FUNCTION_BLOCK PS_PackML_StateMachine_Auto
VAR_INPUT
	Start				: BOOL;
	Hold				: BOOL;
	UnHold				: BOOL;
	Suspend				: BOOL;
	UnSuspend			: BOOL;
	Abort				: BOOL;
	Stop				: BOOL;
	Complete			: BOOL;
	Clear				: BOOL;
	Reset				: BOOL;
	StateComplete		: BOOL;
END_VAR
VAR_OUTPUT
	Status				: WORD;

	ST_Starting			: BOOL;
	ST_Completing		: BOOL;
	ST_Resetting		: BOOL;
	ST_Holding			: BOOL;
	ST_UnHolding		: BOOL;
	ST_Suspending		: BOOL;
	ST_UnSuspending		: BOOL;
	ST_Clearing			: BOOL;
	ST_Stopping			: BOOL;
	ST_Aborting			: BOOL;

	(* State Complete*)
	ST_Execute			: BOOL;
	ST_Complete			: BOOL;
	ST_Idle				: BOOL;
	ST_Held				: BOOL;
	ST_Suspended		: BOOL;
	ST_Stopped			: BOOL;
	ST_Aborted			: BOOL;

	(* additional *)
	Error				: BOOL;
	ErrorID				: DWORD;
	ePMLState			: E_PMLState := E_PMLState.IDLE;
END_VAR
VAR
	ePMLStatePrev		: E_PMLState;
	bStateChange		: BOOL;
	StateCompletePrev	: BOOL;
END_VAR

(* check for state change *)
IF ePMLStatePrev <> ePMLState THEN
	ePMLStatePrev 	:= ePMLState;
	bStateChange	:= TRUE;
ELSE
	bStateChange	:= FALSE;
END_IF


(* change to new state if requested *)
CASE ePMLState OF
	E_PMLState.UNDEFINED:
				(* undefined state *)
				IF bStateChange THEN
					(* transient state *)
					ST_Starting		:= FALSE;
					ST_Completing	:= FALSE;
					ST_Resetting	:= FALSE;
					ST_Holding		:= FALSE;
					ST_UnHolding	:= FALSE;
					ST_Suspending	:= FALSE;
					ST_UnSuspending	:= FALSE;
					ST_Clearing		:= FALSE;
					ST_Stopping		:= FALSE;
					ST_Aborting		:= FALSE;
		
					(* final state *)
					ST_Execute		:= FALSE;
					ST_Complete		:= FALSE;
					ST_Idle			:= FALSE;
					ST_Held			:= FALSE;
					ST_Suspended	:= FALSE;
					ST_Stopped		:= FALSE;
					ST_Aborted		:= FALSE;
				END_IF
		
				IF Abort THEN
					ePMLState 		:= E_PMLState.ABORTING;
					ST_Aborting		:= TRUE;
				ELSIF Stop THEN
					ePMLState 		:= E_PMLState.STOPPING;
					ST_Stopping		:= TRUE;
				END_IF


	E_PMLState.IDLE:
				(* final state *)
		
				IF bStateChange THEN
					(* transient state *)
					ST_Starting		:= FALSE;
					ST_Completing	:= FALSE;
					ST_Resetting	:= FALSE;
					ST_Holding		:= FALSE;
					ST_UnHolding	:= FALSE;
					ST_Suspending	:= FALSE;
					ST_UnSuspending	:= FALSE;
					ST_Clearing		:= FALSE;
					ST_Stopping		:= FALSE;
					ST_Aborting		:= FALSE;
		
					(* final state *)
					ST_Execute		:= FALSE;
					ST_Complete		:= FALSE;
					ST_Idle			:= TRUE;
					ST_Held			:= FALSE;
					ST_Suspended	:= FALSE;
					ST_Stopped		:= FALSE;
					ST_Aborted		:= FALSE;
				END_IF
		
				IF Abort THEN
					ePMLState 		:= E_PMLState.ABORTING;
					ST_Idle			:= FALSE;
					ST_Aborting		:= TRUE;
				ELSIF Stop THEN
					ePMLState 		:= E_PMLState.STOPPING;
					ST_Idle			:= FALSE;
					ST_Stopping		:= TRUE;
				ELSIF Start THEN
					ePMLState 		:= E_PMLState.STARTING;
					ST_Idle			:= FALSE;
					ST_Starting		:= TRUE;
				END_IF


	E_PMLState.STARTING:
				(* transient state *)
		
				IF bStateChange THEN
					(* transient state *)
					ST_Starting		:= TRUE;
					ST_Completing	:= FALSE;
					ST_Resetting	:= FALSE;
					ST_Holding		:= FALSE;
					ST_UnHolding	:= FALSE;
					ST_Suspending	:= FALSE;
					ST_UnSuspending	:= FALSE;
					ST_Clearing		:= FALSE;
					ST_Stopping		:= FALSE;
					ST_Aborting		:= FALSE;
		
					(* final state *)
					ST_Execute		:= FALSE;
					ST_Complete		:= FALSE;
					ST_Idle			:= FALSE;
					ST_Held			:= FALSE;
					ST_Suspended	:= FALSE;
					ST_Stopped		:= FALSE;
					ST_Aborted		:= FALSE;
				END_IF
		
				IF Abort THEN
					ePMLState 		:= E_PMLState.ABORTING;
					ST_Starting		:= FALSE;
					ST_Aborting		:= TRUE;
				ELSIF Stop THEN
					ePMLState 		:= E_PMLState.STOPPING;
					ST_Starting		:= FALSE;
					ST_Stopping		:= TRUE;
				ELSIF StateComplete AND NOT StateCompletePrev THEN
					ePMLState 		:= E_PMLState.EXECUTE;
					StateCompletePrev := StateComplete;
					ST_Starting		:= FALSE;
					ST_Execute		:= TRUE;
				END_IF


	E_PMLState.EXECUTE:
				(* final state *)
		
				IF bStateChange THEN
					(* transient state *)
					ST_Starting		:= FALSE;
					ST_Completing	:= FALSE;
					ST_Resetting	:= FALSE;
					ST_Holding		:= FALSE;
					ST_UnHolding	:= FALSE;
					ST_Suspending	:= FALSE;
					ST_UnSuspending	:= FALSE;
					ST_Clearing		:= FALSE;
					ST_Stopping		:= FALSE;
					ST_Aborting		:= FALSE;
		
					(* final state *)
					ST_Execute		:= TRUE;
					ST_Complete		:= FALSE;
					ST_Idle			:= FALSE;
					ST_Held			:= FALSE;
					ST_Suspended	:= FALSE;
					ST_Stopped		:= FALSE;
					ST_Aborted		:= FALSE;
				END_IF
		
				IF Abort THEN
					ePMLState 		:= E_PMLState.ABORTING;
					ST_Execute		:= FALSE;
					ST_Aborting		:= TRUE;
				ELSIF Stop THEN
					ePMLState 		:= E_PMLState.STOPPING;
					ST_Execute		:= FALSE;
					ST_Stopping		:= TRUE;
				ELSIF Suspend THEN
					ePMLState 		:= E_PMLState.SUSPENDING;
					ST_Execute		:= FALSE;
					ST_Suspending	:= TRUE;
				ELSIF Hold THEN
					ePMLState 		:= E_PMLState.HOLDING;
					ST_Execute		:= FALSE;
					ST_Holding		:= TRUE;
				ELSIF Complete THEN
					ePMLState 		:= E_PMLState.COMPLETING;
					ST_Execute		:= FALSE;
					ST_Completing	:= TRUE;
				END_IF


	E_PMLState.COMPLETING:
				(* transient state *)
		
				IF bStateChange THEN
					(* transient state *)
					ST_Starting		:= FALSE;
					ST_Completing	:= TRUE;
					ST_Resetting	:= FALSE;
					ST_Holding		:= FALSE;
					ST_UnHolding	:= FALSE;
					ST_Suspending	:= FALSE;
					ST_UnSuspending	:= FALSE;
					ST_Clearing		:= FALSE;
					ST_Stopping		:= FALSE;
					ST_Aborting		:= FALSE;
		
					(* final state *)
					ST_Execute		:= FALSE;
					ST_Complete		:= FALSE;
					ST_Idle			:= FALSE;
					ST_Held			:= FALSE;
					ST_Suspended	:= FALSE;
					ST_Stopped		:= FALSE;
					ST_Aborted		:= FALSE;
				END_IF
		
				IF Abort THEN
					ePMLState 		:= E_PMLState.ABORTING;
					ST_Completing	:= FALSE;
					ST_Aborting		:= TRUE;
				ELSIF Stop THEN
					ePMLState 		:= E_PMLState.STOPPING;
					ST_Completing	:= FALSE;
					ST_Stopping		:= TRUE;
				ELSIF StateComplete AND NOT StateCompletePrev THEN
					ePMLState 		:= E_PMLState.COMPLETE;
					StateCompletePrev := StateComplete;
					ST_Completing	:= FALSE;
					ST_Complete		:= TRUE;
				END_IF


	E_PMLState.COMPLETE:
				(* final state *)
		
				IF bStateChange THEN
					(* transient state *)
					ST_Starting		:= FALSE;
					ST_Completing	:= FALSE;
					ST_Resetting	:= FALSE;
					ST_Holding		:= FALSE;
					ST_UnHolding	:= FALSE;
					ST_Suspending	:= FALSE;
					ST_UnSuspending	:= FALSE;
					ST_Clearing		:= FALSE;
					ST_Stopping		:= FALSE;
					ST_Aborting		:= FALSE;
		
					(* final state *)
					ST_Execute		:= FALSE;
					ST_Complete		:= TRUE;
					ST_Idle			:= FALSE;
					ST_Held			:= FALSE;
					ST_Suspended	:= FALSE;
					ST_Stopped		:= FALSE;
					ST_Aborted		:= FALSE;
				END_IF
		
				IF Abort THEN
					ePMLState 		:= E_PMLState.ABORTING;
					ST_Complete		:= FALSE;
					ST_Aborting		:= TRUE;
				ELSIF Stop THEN
					ePMLState 		:= E_PMLState.STOPPING;
					ST_Complete		:= FALSE;
					ST_Stopping		:= TRUE;
				ELSIF Reset THEN
					ePMLState 		:= E_PMLState.RESETTING;
					ST_Complete		:= FALSE;
					ST_Resetting	:= TRUE;
				END_IF


	E_PMLState.RESETTING:
				(* transient state *)
		
				IF bStateChange THEN
					(* transient state *)
					ST_Starting		:= FALSE;
					ST_Completing	:= FALSE;
					ST_Resetting	:= TRUE;
					ST_Holding		:= FALSE;
					ST_UnHolding	:= FALSE;
					ST_Suspending	:= FALSE;
					ST_UnSuspending	:= FALSE;
					ST_Clearing		:= FALSE;
					ST_Stopping		:= FALSE;
					ST_Aborting		:= FALSE;
		
					(* final state *)
					ST_Execute		:= FALSE;
					ST_Complete		:= FALSE;
					ST_Idle			:= FALSE;
					ST_Held			:= FALSE;
					ST_Suspended	:= FALSE;
					ST_Stopped		:= FALSE;
					ST_Aborted		:= FALSE;
				END_IF
		
				IF Abort THEN
					ePMLState 		:= E_PMLState.ABORTING;
					ST_Resetting	:= FALSE;
					ST_Aborting		:= TRUE;
				ELSIF Stop THEN
					ePMLState 		:= E_PMLState.STOPPING;
					ST_Resetting	:= FALSE;
					ST_Stopping		:= TRUE;
				ELSIF StateComplete THEN
					ePMLState 		:= E_PMLState.IDLE;
					StateCompletePrev := StateComplete;
					ST_Resetting	:= FALSE;
					ST_Idle			:= TRUE;
				END_IF


	E_PMLState.HOLDING:
				(* transient state *)
		
				IF bStateChange THEN
					(* transient state *)
					ST_Starting		:= FALSE;
					ST_Completing	:= FALSE;
					ST_Resetting	:= FALSE;
					ST_Holding		:= TRUE;
					ST_UnHolding	:= FALSE;
					ST_Suspending	:= FALSE;
					ST_UnSuspending	:= FALSE;
					ST_Clearing		:= FALSE;
					ST_Stopping		:= FALSE;
					ST_Aborting		:= FALSE;
		
					(* final state *)
					ST_Execute		:= FALSE;
					ST_Complete		:= FALSE;
					ST_Idle			:= FALSE;
					ST_Held			:= FALSE;
					ST_Suspended	:= FALSE;
					ST_Stopped		:= FALSE;
					ST_Aborted		:= FALSE;
				END_IF
		
				IF Abort THEN
					ePMLState 		:= E_PMLState.ABORTING;
					ST_Holding		:= FALSE;
					ST_Aborting		:= TRUE;
				ELSIF Stop THEN
					ePMLState 		:= E_PMLState.STOPPING;
					ST_Holding		:= FALSE;
					ST_Stopping		:= TRUE;
				ELSIF StateComplete AND NOT StateCompletePrev THEN
					ePMLState 		:= E_PMLState.HELD;
					StateCompletePrev := StateComplete;
					ST_Holding		:= FALSE;
					ST_Held			:= TRUE;
				END_IF


	E_PMLState.HELD:
				(* final state *)

				IF bStateChange THEN
					(* transient state *)
					ST_Starting		:= FALSE;
					ST_Completing	:= FALSE;
					ST_Resetting	:= FALSE;
					ST_Holding		:= FALSE;
					ST_UnHolding	:= FALSE;
					ST_Suspending	:= FALSE;
					ST_UnSuspending	:= FALSE;
					ST_Clearing		:= FALSE;
					ST_Stopping		:= FALSE;
					ST_Aborting		:= FALSE;
		
					(* final state *)
					ST_Execute		:= FALSE;
					ST_Complete		:= FALSE;
					ST_Idle			:= FALSE;
					ST_Held			:= TRUE;
					ST_Suspended	:= FALSE;
					ST_Stopped		:= FALSE;
					ST_Aborted		:= FALSE;
				END_IF
		
				IF Abort THEN
					ePMLState 		:= E_PMLState.ABORTING;
					ST_Held			:= FALSE;
					ST_Aborting		:= TRUE;
				ELSIF Stop THEN
					ePMLState 		:= E_PMLState.STOPPING;
					ST_Held			:= FALSE;
					ST_Stopping		:= TRUE;
				ELSIF UnHold THEN
					ePMLState 		:= E_PMLState.UNHOLDING;
					ST_Held			:= FALSE;
					ST_UnHolding	:= TRUE;
				END_IF


	E_PMLState.UNHOLDING:
				(* transient state *)
		
				IF bStateChange THEN
					(* transient state *)
					ST_Starting		:= FALSE;
					ST_Completing	:= FALSE;
					ST_Resetting	:= FALSE;
					ST_Holding		:= FALSE;
					ST_UnHolding	:= TRUE;
					ST_Suspending	:= FALSE;
					ST_UnSuspending	:= FALSE;
					ST_Clearing		:= FALSE;
					ST_Stopping		:= FALSE;
					ST_Aborting		:= FALSE;
		
					(* final state *)
					ST_Execute		:= FALSE;
					ST_Complete		:= FALSE;
					ST_Idle			:= FALSE;
					ST_Held			:= FALSE;
					ST_Suspended	:= FALSE;
					ST_Stopped		:= FALSE;
					ST_Aborted		:= FALSE;
				END_IF
		
				IF Abort THEN
					ePMLState 		:= E_PMLState.ABORTING;
					ST_UnHolding	:= FALSE;
					ST_Aborting		:= TRUE;
				ELSIF Stop THEN
					ePMLState 		:= E_PMLState.STOPPING;
					ST_UnHolding	:= FALSE;
					ST_Stopping		:= TRUE;
				ELSIF StateComplete AND NOT StateCompletePrev THEN
					ePMLState 		:= E_PMLState.EXECUTE;
					StateCompletePrev := StateComplete;
					ST_UnHolding	:= FALSE;
					ST_Execute		:= TRUE;
				END_IF


	E_PMLState.SUSPENDING:
				(* transient state *)
		
				IF bStateChange THEN
					(* transient state *)
					ST_Starting		:= FALSE;
					ST_Completing	:= FALSE;
					ST_Resetting	:= FALSE;
					ST_Holding		:= FALSE;
					ST_UnHolding	:= FALSE;
					ST_Suspending	:= TRUE;
					ST_UnSuspending	:= FALSE;
					ST_Clearing		:= FALSE;
					ST_Stopping		:= FALSE;
					ST_Aborting		:= FALSE;
		
					(* final state *)
					ST_Execute		:= FALSE;
					ST_Complete		:= FALSE;
					ST_Idle			:= FALSE;
					ST_Held			:= FALSE;
					ST_Suspended	:= FALSE;
					ST_Stopped		:= FALSE;
					ST_Aborted		:= FALSE;
				END_IF
		
				IF Abort THEN
					ePMLState 		:= E_PMLState.ABORTING;
					ST_Suspending	:= FALSE;
					ST_Aborting		:= TRUE;
				ELSIF Stop THEN
					ePMLState 		:= E_PMLState.STOPPING;
					ST_Suspending	:= FALSE;
					ST_Stopping		:= TRUE;
				ELSIF StateComplete AND NOT StateCompletePrev THEN
					ePMLState 		:= E_PMLState.SUSPENDED;
					StateCompletePrev := StateComplete;
					ST_Suspending	:= FALSE;
					ST_Suspended	:= TRUE;
				END_IF


	E_PMLState.SUSPENDED:
				(* final state *)
		
				IF bStateChange THEN
					(* transient state *)
					ST_Starting		:= FALSE;
					ST_Completing	:= FALSE;
					ST_Resetting	:= FALSE;
					ST_Holding		:= FALSE;
					ST_UnHolding	:= FALSE;
					ST_Suspending	:= FALSE;
					ST_UnSuspending	:= FALSE;
					ST_Clearing		:= FALSE;
					ST_Stopping		:= FALSE;
					ST_Aborting		:= FALSE;
		
					(* final state *)
					ST_Execute		:= FALSE;
					ST_Complete		:= FALSE;
					ST_Idle			:= FALSE;
					ST_Held			:= FALSE;
					ST_Suspended	:= TRUE;
					ST_Stopped		:= FALSE;
					ST_Aborted		:= FALSE;
				END_IF
		
				IF Abort THEN
					ePMLState 		:= E_PMLState.ABORTING;
					ST_Suspended	:= FALSE;
					ST_Aborting		:= TRUE;
				ELSIF Stop THEN
					ePMLState 		:= E_PMLState.STOPPING;
					ST_Suspended	:= FALSE;
					ST_Stopping		:= TRUE;
				ELSIF UnSuspend THEN
					ePMLState 		:= E_PMLState.UNSUSPENDING;
					ST_Suspended	:= FALSE;
					ST_UnSuspending	:= TRUE;
				END_IF


	E_PMLState.UNSUSPENDING:
				(* transient state *)
		
				IF bStateChange THEN
					(* transient state *)
					ST_Starting		:= FALSE;
					ST_Completing	:= FALSE;
					ST_Resetting	:= FALSE;
					ST_Holding		:= FALSE;
					ST_UnHolding	:= FALSE;
					ST_Suspending	:= FALSE;
					ST_UnSuspending	:= TRUE;
					ST_Clearing		:= FALSE;
					ST_Stopping		:= FALSE;
					ST_Aborting		:= FALSE;
		
					(* final state *)
					ST_Execute		:= FALSE;
					ST_Complete		:= FALSE;
					ST_Idle			:= FALSE;
					ST_Held			:= FALSE;
					ST_Suspended	:= FALSE;
					ST_Stopped		:= FALSE;
					ST_Aborted		:= FALSE;
				END_IF
		
				IF Abort THEN
					ePMLState 		:= E_PMLState.ABORTING;
					ST_UnSuspending	:= FALSE;
					ST_Aborting		:= TRUE;
				ELSIF Stop THEN
					ePMLState 		:= E_PMLState.STOPPING;
					ST_UnSuspending	:= FALSE;
					ST_Stopping		:= TRUE;
				ELSIF StateComplete AND NOT StateCompletePrev THEN
					ePMLState 		:= E_PMLState.EXECUTE;
					StateCompletePrev := StateComplete;
					ST_UnSuspending	:= FALSE;
					ST_Execute		:= TRUE;
				END_IF


	E_PMLState.STOPPING:
				(* transient state *)
		
				IF bStateChange THEN
					(* transient state *)
					ST_Starting		:= FALSE;
					ST_Completing	:= FALSE;
					ST_Resetting	:= FALSE;
					ST_Holding		:= FALSE;
					ST_UnHolding	:= FALSE;
					ST_Suspending	:= FALSE;
					ST_UnSuspending	:= FALSE;
					ST_Clearing		:= FALSE;
					ST_Stopping		:= TRUE;
					ST_Aborting		:= FALSE;
		
					(* final state *)
					ST_Execute		:= FALSE;
					ST_Complete		:= FALSE;
					ST_Idle			:= FALSE;
					ST_Held			:= FALSE;
					ST_Suspended	:= FALSE;
					ST_Stopped		:= FALSE;
					ST_Aborted		:= FALSE;
				END_IF
		
				IF Abort THEN
					ePMLState 		:= E_PMLState.ABORTING;
					ST_Stopping		:= FALSE;
					ST_Aborting		:= TRUE;
				ELSIF StateComplete AND NOT StateCompletePrev THEN
					ePMLState 		:= E_PMLState.STOPPED;
					StateCompletePrev := StateComplete;
					ST_Stopping		:= FALSE;
					ST_Stopped		:= TRUE;
				END_IF
				

	E_PMLState.STOPPED:
				(* final state *)
		
				IF bStateChange THEN
					(* transient state *)
					ST_Starting		:= FALSE;
					ST_Completing	:= FALSE;
					ST_Resetting	:= FALSE;
					ST_Holding		:= FALSE;
					ST_UnHolding	:= FALSE;
					ST_Suspending	:= FALSE;
					ST_UnSuspending	:= FALSE;
					ST_Clearing		:= FALSE;
					ST_Stopping		:= FALSE;
					ST_Aborting		:= FALSE;
		
					(* final state *)
					ST_Execute		:= FALSE;
					ST_Complete		:= FALSE;
					ST_Idle			:= FALSE;
					ST_Held			:= FALSE;
					ST_Suspended	:= FALSE;
					ST_Stopped		:= TRUE;
					ST_Aborted		:= FALSE;
				END_IF
		
				IF Abort THEN
					ePMLState 		:= E_PMLState.ABORTING;
					ST_Stopped		:= FALSE;
					ST_Aborting		:= TRUE;
				ELSIF Reset THEN
					ePMLState 		:= E_PMLState.RESETTING;
					ST_Stopped		:= FALSE;
					ST_Resetting	:= TRUE;
				END_IF


	E_PMLState.ABORTING:
				(* transient state *)
		
				IF bStateChange THEN
					(* transient state *)
					ST_Starting		:= FALSE;
					ST_Completing	:= FALSE;
					ST_Resetting	:= FALSE;
					ST_Holding		:= FALSE;
					ST_UnHolding	:= FALSE;
					ST_Suspending	:= FALSE;
					ST_UnSuspending	:= FALSE;
					ST_Clearing		:= FALSE;
					ST_Stopping		:= FALSE;
					ST_Aborting		:= TRUE;
		
					(* final state *)
					ST_Execute		:= FALSE;
					ST_Complete		:= FALSE;
					ST_Idle			:= FALSE;
					ST_Held			:= FALSE;
					ST_Suspended	:= FALSE;
					ST_Stopped		:= FALSE;
					ST_Aborted		:= FALSE;
				END_IF
		
				IF StateComplete AND NOT StateCompletePrev THEN
					ePMLState 		:= E_PMLState.ABORTED;
					StateCompletePrev := StateComplete;
					ST_Aborting		:= FALSE;
					ST_Aborted		:= TRUE;
				END_IF


	E_PMLState.ABORTED:
				(* final state *)
		
				IF bStateChange THEN
					(* transient state *)
					ST_Starting		:= FALSE;
					ST_Completing	:= FALSE;
					ST_Resetting	:= FALSE;
					ST_Holding		:= FALSE;
					ST_UnHolding	:= FALSE;
					ST_Suspending	:= FALSE;
					ST_UnSuspending	:= FALSE;
					ST_Clearing		:= FALSE;
					ST_Stopping		:= FALSE;
					ST_Aborting		:= FALSE;
		
					(* final state *)
					ST_Execute		:= FALSE;
					ST_Complete		:= FALSE;
					ST_Idle			:= FALSE;
					ST_Held			:= FALSE;
					ST_Suspended	:= FALSE;
					ST_Stopped		:= FALSE;
					ST_Aborted		:= TRUE;
				END_IF
		
				IF Clear THEN
					ePMLState 		:= E_PMLState.CLEARING;
					ST_Aborted		:= FALSE;
					ST_Clearing		:= TRUE;
				END_IF


	E_PMLState.CLEARING:
				(* transient state *)
		
				IF bStateChange THEN
					(* transient state *)
					ST_Starting		:= FALSE;
					ST_Completing	:= FALSE;
					ST_Resetting	:= FALSE;
					ST_Holding		:= FALSE;
					ST_UnHolding	:= FALSE;
					ST_Suspending	:= FALSE;
					ST_UnSuspending	:= FALSE;
					ST_Clearing		:= TRUE;
					ST_Stopping		:= FALSE;
					ST_Aborting		:= FALSE;
		
					(* final state *)
					ST_Execute		:= FALSE;
					ST_Complete		:= FALSE;
					ST_Idle			:= FALSE;
					ST_Held			:= FALSE;
					ST_Suspended	:= FALSE;
					ST_Stopped		:= FALSE;
					ST_Aborted		:= FALSE;
				END_IF
		
				IF Abort THEN
					ePMLState 		:= E_PMLState.ABORTING;
					ST_Stopped		:= FALSE;
					ST_Aborting		:= TRUE;
				ELSIF StateComplete AND NOT StateCompletePrev THEN
					ePMLState 		:= E_PMLState.STOPPED;
					StateCompletePrev := StateComplete;
					ST_Clearing		:= FALSE;
					ST_Stopped		:= TRUE;
				END_IF

END_CASE

(* auto clear with StateComplete = FALSE *)
StateCompletePrev := StateCompletePrev AND StateComplete;

END_FUNCTION_BLOCK
